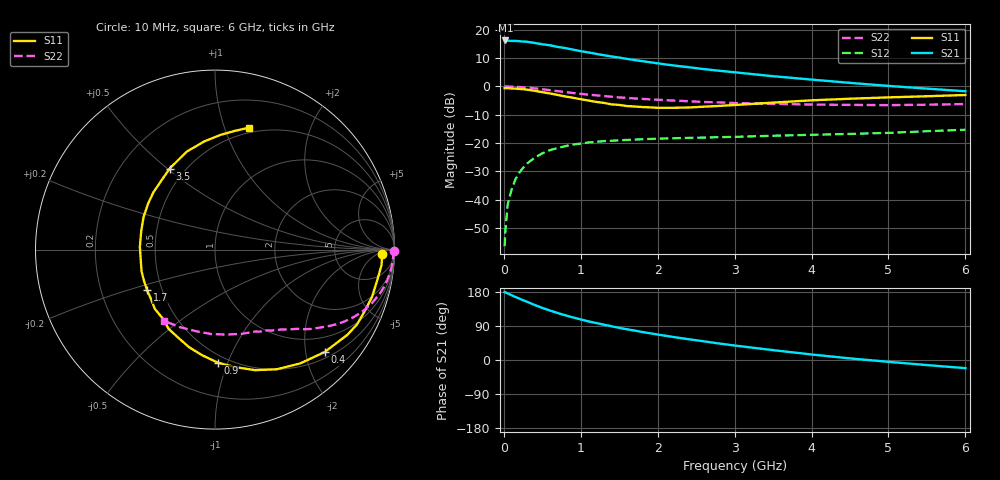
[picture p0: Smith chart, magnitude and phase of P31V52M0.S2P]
! SIEMENS Small Signal Semiconductors
! BFP181
! Si NPN RF Bipolar Junction Transistor in SOT143
! VCE = 1.5 V  IC = 2 mA
! Common Emitter S-Parameters:  March  1996
# GHz  S  MA  R  50
!  f  S11  S21  S12  S22
! GHz  MAG  ANG  MAG  ANG  MAG  ANG  MAG  ANG
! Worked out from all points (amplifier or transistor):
!   36 points, 10 MHz to 6 GHz, reference 50 ohm
!   highest |S21| = 16.3 dB at 20 MHz (marker M1)
!   |S21| within 3 dB of that: start of sweep to 854.6 MHz
!   unconditionally stable (mu >= 1): 2.365 GHz to end of sweep
!   at 250 MHz: K = 0.13, MSG = 22.3 dB, |S12| = -28.8 dB
!   at 1.4 GHz: K = 0.67, MSG = 14.9 dB, |S12| = -19.2 dB
!   at 6 GHz: K = 1.16, MAG = 4.4 dB, |S12| = -15.3 dB
!   S11 on the Smith chart (normalised r, x): 10 MHz: 25, -8; 400 MHz: 0.63, -2.39; 900 MHz: 0.44, -0.92; 1.7 GHz: 0.41, -0.23; 3.5 GHz: 0.41, +0.51; 6 GHz: 0.45, +1.22
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0.01  0.9303 -1.4  6.451 179.3  0.0015 86.5  0.9976 -0.4
0.02  0.9319 -2.5  6.494 178.7  0.0028 87.0  0.9923 -1.0
0.05  0.9318 -5.3  6.449 175.5  0.0082 89.8  0.9937 -2.5
0.15  0.9138 -16.7  6.371 166.5  0.0227 79.0  0.9836 -7.6
0.25  0.8947 -27.7  6.212 157.7  0.0364 73.4  0.9648 -12.4
0.3  0.877 -32.8  6.158 153.9  0.0431 70.2  0.9521 -14.7
0.4  0.8359 -43.1  5.873 145.2  0.055 64.5  0.9233 -18.9
0.5  0.7921 -53.2  5.561 137.5  0.0656 58.8  0.8917 -22.7
0.6  0.7503 -62.7  5.332 130.5  0.0749 54.1  0.858 -26.1
0.7  0.7078 -71.6  4.995 124.0  0.0814 49.9  0.8243 -29.1
0.8  0.6641 -80.3  4.758 117.8  0.0881 45.9  0.7942 -31.6
0.9  0.6303 -88.5  4.468 112.3  0.0938 42.6  0.765 -33.8
1.1  0.563 -104.8  3.99 101.9  0.1021 36.8  0.7155 -37.7
1.4  0.4813 -127.4  3.385 89.0  0.1097 30.4  0.6572 -42.5
1.7  0.4411 -149.2  2.923 77.6  0.1149 26.4  0.6128 -46.4
1.9  0.4266 -163.6  2.677 70.6  0.1179 23.8  0.5904 -48.9
2.2  0.4189 177.7  2.352 60.8  0.1209 21.4  0.5623 -52.8
2.8  0.4523 145.5  1.893 43.5  0.1269 17.6  0.5222 -61.1
3.5  0.5174 119.3  1.515 26.0  0.1344 15.1  0.4926 -72.3
4.5  0.606 95.6  1.155 4.2  0.1448 11.5  0.4711 -92.6
5.5  0.6702 80.6  0.914 -13.4  0.1614 10.1  0.4744 -114.5
6  0.7055 74.4  0.821 -21.5  0.1716 8.0  0.4886 -125.7
